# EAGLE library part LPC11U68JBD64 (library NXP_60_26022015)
32-bit ARM Cortex-M0+ microcontroller; up to 256 kB flash and 36 kB SRAM; 4 kB EEPROM; USB; 12-bit ADC The LPC11U6x are an ARM Cortex-M0+ based, low-cost 32-bit MCU family operating at CPU frequencies of up to 50 MHz. The LPC11U6x support up to 256 kB of flash memory, a 4 kB EEPROM, and 36 kB of SRAM. The ARM Cortex-M0+ is an easy-to-use, energy-efficient core using a two-stage pipeline and fast single-cycle I/O access. The peripheral complement of the LPC11U6x includes a DMA controller, a CRC engine, one full-speed USB device controller with XTAL-less low-speed mode, two I2C-bus interfaces, up to five USARTs, two SSP interfaces, PWM/timer subsystem with six configurable multi-purpose timers, a Real-Time Clock, one 12-bit ADC, temperature sensor, function-configurable I/O ports, and up to 80 general-purpose I/O pins. AAL Eindhoven MK
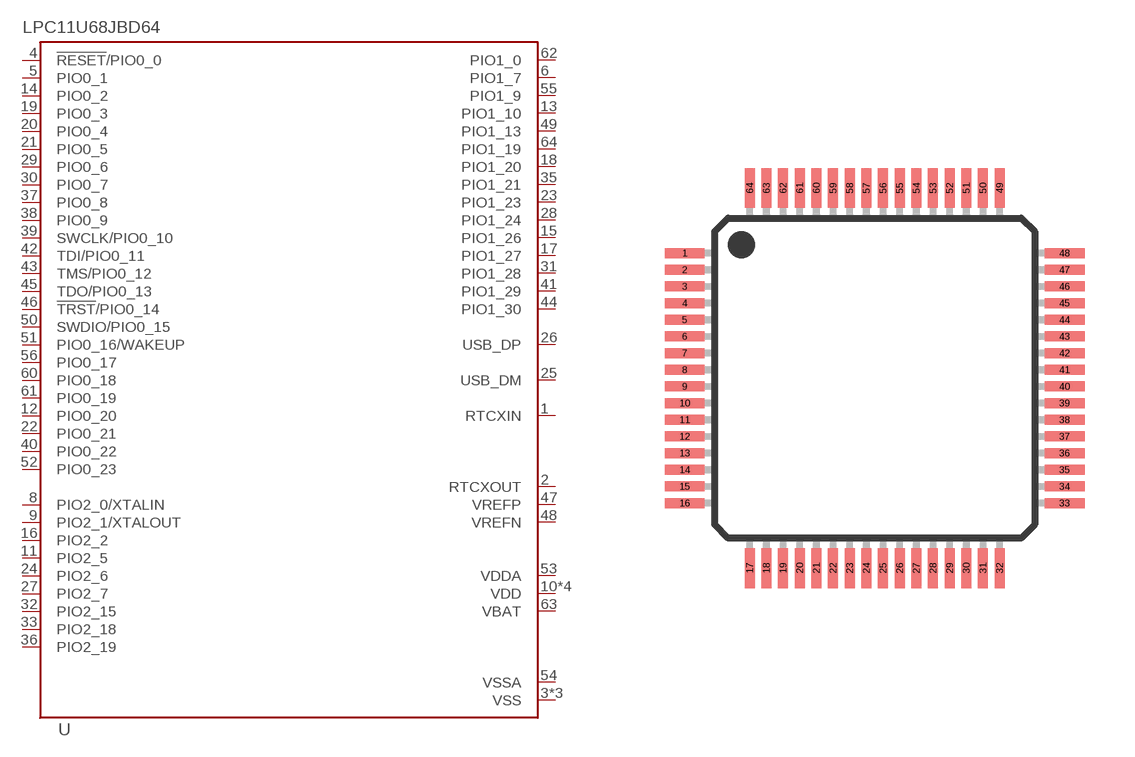
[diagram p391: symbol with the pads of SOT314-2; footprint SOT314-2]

Designator prefix U

## LPC11U68JBD64  [SOT314-2]
1  RTCXIN
2  RTCXOUT
3  VSS
4  !RESET!/PIO0_0
5  PIO0_1
6  PIO1_7
7  VSS
8  PIO2_0/XTALIN
9  PIO2_1/XTALOUT
10  VDD
11  PIO2_5
12  PIO0_20
13  PIO1_10
14  PIO0_2
15  PIO1_26
16  PIO2_2
17  PIO1_27
18  PIO1_20
19  PIO0_3
20  PIO0_4
21  PIO0_5
22  PIO0_21
23  PIO1_23
24  PIO2_6
25  USB_DM
26  USB_DP
27  PIO2_7
28  PIO1_24
29  PIO0_6
30  PIO0_7
31  PIO1_28
32  PIO2_15
33  PIO2_18
34  VDD
35  PIO1_21
36  PIO2_19
37  PIO0_8
38  PIO0_9
39  SWCLK/PIO0_10
40  PIO0_22
41  PIO1_29
42  TDI/PIO0_11
43  TMS/PIO0_12
44  PIO1_30
45  TDO/PIO0_13
46  !TRST!/PIO0_14
47  VREFP
48  VREFN
49  PIO1_13
50  SWDIO/PIO0_15
51  PIO0_16/WAKEUP
52  PIO0_23
53  VDDA
54  VSSA
55  PIO1_9
56  PIO0_17
57  VSS
58  VDD
59  VDD
60  PIO0_18
61  PIO0_19
62  PIO1_0
63  VBAT
64  PIO1_19

## Footprint SOT314-2 (pad centres in mm)
SOT314-2 LQFP64: plastic low profile quad flat package; 64 leads; body 10 x 10 x 1.4 mm JEDEC: MS-026 IEC: 136E10
smd 1.2 x 0.3: 1 -5.7,3.75; 2 -5.7,3.25; 3 -5.7,2.75; 4 -5.7,2.25; 5 -5.7,1.75; 6 -5.7,1.25; 7 -5.7,0.75; 8 -5.7,0.25; 9 -5.7,-0.25; 10 -5.7,-0.75; 11 -5.7,-1.25; 12 -5.7,-1.75; 13 -5.7,-2.25; 14 -5.7,-2.75; 15 -5.7,-3.25; 16 -5.7,-3.75; 33 5.7,-3.75; 34 5.7,-3.25; 35 5.7,-2.75; 36 5.7,-2.25; 37 5.7,-1.75; 38 5.7,-1.25; 39 5.7,-0.75; 40 5.7,-0.25; 41 5.7,0.25; 42 5.7,0.75; 43 5.7,1.25; 44 5.7,1.75; 45 5.7,2.25; 46 5.7,2.75; 47 5.7,3.25; 48 5.7,3.75
smd 0.3 x 1.2: 17 -3.75,-5.7; 18 -3.25,-5.7; 19 -2.75,-5.7; 20 -2.25,-5.7; 21 -1.75,-5.7; 22 -1.25,-5.7; 23 -0.75,-5.7; 24 -0.25,-5.7; 25 0.25,-5.7; 26 0.75,-5.7; 27 1.25,-5.7; 28 1.75,-5.7; 29 2.25,-5.7; 30 2.75,-5.7; 31 3.25,-5.7; 32 3.75,-5.7; 49 3.75,5.7; 50 3.25,5.7; 51 2.75,5.7; 52 2.25,5.7; 53 1.75,5.7; 54 1.25,5.7; 55 0.75,5.7; 56 0.25,5.7; 57 -0.25,5.7; 58 -0.75,5.7; 59 -1.25,5.7; 60 -1.75,5.7; 61 -2.25,5.7; 62 -2.75,5.7; 63 -3.25,5.7; 64 -3.75,5.7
